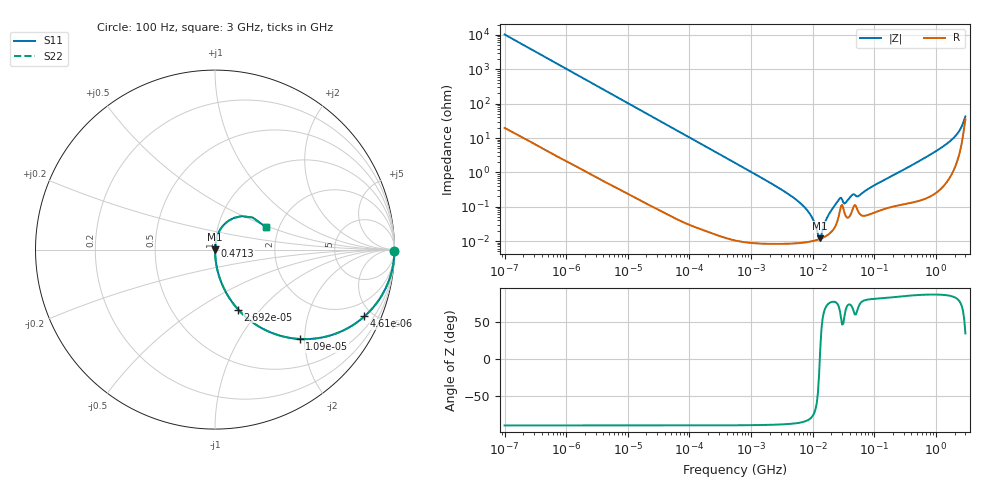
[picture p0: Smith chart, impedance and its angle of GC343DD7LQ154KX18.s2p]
!Murata Part Number: GC343DD7LQ154KX18
!These Parameters are Measured in Series Mode Connection
!Data Generated on Jan 08, 2026
!  o--ll--o
!Port1  Port2
!  o------o
!Operation Temp=25[degC], DC Bias Voltage=0[V]
!Freq. Start=100[Hz] Stop=3[GHz] 401[Steps]
# Hz S RI R 50
!Freq.(Hz) S11(Real) S11(Imag) S21(Real) S21(Imag) S12(Real) S12(Imag) S22(Real) S22(Imag)
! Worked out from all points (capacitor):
!   401 points, 100 Hz to 3 GHz, reference 50 ohm
!   read as one part in series: C = 155 nF near 109 Hz
!   lowest |Z| = 12 mohm at 13.24 MHz (marker M1)
!   series resonance near 13.03 MHz, so ESL is about 960 pH
!   S11 on the Smith chart (normalised r, x): 100 Hz: open; 4.61 kHz: 1.01, -4.47; 10.9 kHz: 1.00, -1.89; 26.92 kHz: 1.00, -0.77; 471.3 MHz: 1.00, +0.04; 3 GHz: 1.70, +0.48
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100  0.9999 -0.00974  0.000114 0.00974  0.000114 0.00974  0.9999 -0.00974
1788  0.9704 -0.1684  0.0296 0.1684  0.0296 0.1684  0.9704 -0.1684
4610  0.8329 -0.372  0.1671 0.372  0.1671 0.372  0.8329 -0.372
10902  0.4729 -0.4981  0.5271 0.4981  0.5271 0.4981  0.4729 -0.4981
26919  0.1291 -0.3341  0.8709 0.3341  0.8709 0.3341  0.1291 -0.3341
31977  0.0953 -0.2923  0.9047 0.2923  0.9047 0.2923  0.0953 -0.2923
102221  0.0104 -0.1002  0.9896 0.1002  0.9896 0.1002  0.0104 -0.1002
547723  0.000462 -0.0189  0.9995 0.0189  0.9995 0.0189  0.000462 -0.0189
4711951  8.89e-05 -0.00192  0.9999 0.00192  0.9999 0.00192  8.89e-05 -0.00192
9794414  9.99e-05 -0.000467  0.9999 0.000467  0.9999 0.000467  9.99e-05 -0.000467
1.214626e7  0.000111 -0.000114  0.9999 0.000114  0.9999 0.000114  0.000111 -0.000114
1.323817e7  0.000117 2.63e-05  0.9999 -2.63e-05  0.9999 -2.63e-05  0.000117 2.63e-05
1.789277e7  0.000156 0.000545  0.9998 -0.000545  0.9998 -0.000545  0.000156 0.000545
2.635803e7  0.000524 0.00149  0.9995 -0.00149  0.9995 -0.00149  0.000524 0.00149
3.412477e7  0.000547 0.00119  0.9995 -0.00119  0.9995 -0.00119  0.000547 0.00119
4.418008e7  0.000828 0.00208  0.9992 -0.00208  0.9992 -0.00208  0.000828 0.00208
5.719833e7  0.000637 0.00205  0.9994 -0.00205  0.9994 -0.00205  0.000637 0.00205
1.751444e8  0.001 0.00714  0.999 -0.00714  0.999 -0.00714  0.001 0.00714
4.713361e8  0.00175 0.0187  0.9983 -0.0187  0.9983 -0.0187  0.00175 0.0187
1.642185e9  0.0124 0.0756  0.9876 -0.0756  0.9876 -0.0756  0.0124 0.0756
2.419119e9  0.059 0.1478  0.941 -0.1478  0.941 -0.1478  0.059 0.1478
3e9  0.282 0.1265  0.718 -0.1265  0.718 -0.1265  0.282 0.1265
